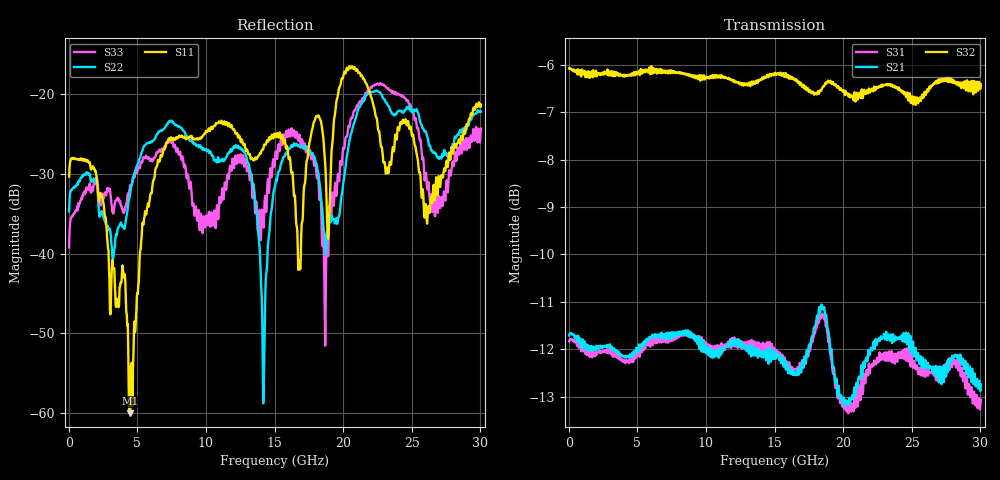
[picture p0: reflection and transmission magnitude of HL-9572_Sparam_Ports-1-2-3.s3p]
# GHZ S RI R 50.0
!; PortSelection: Port_123
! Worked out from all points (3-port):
!   858 points, 35 MHz to 30.03 GHz, reference 50 ohm
!   strongest paths, dB at 35 MHz, 7.525 GHz, 15.05 GHz, 22.54 GHz, 30.03 GHz:
!     S32: -6.1, -6.1, -6.2, -6.5, -6.4
!     S21: -11.7, -11.7, -12.2, -11.8, -12.7
!     S31: -11.8, -11.8, -12.1, -12.2, -13.1
!   lowest |S11| = -60.1 dB at 4.48 GHz (marker M1), VSWR 1.00, Z = 50.1 - j0.0158 ohm
!   |S11| at or under -10 dB: start of sweep to end of sweep
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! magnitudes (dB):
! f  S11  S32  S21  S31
! 35 MHz  -30.3  -6.1  -11.7  -11.8
! 4.48 GHz  -60.1  -6.2  -12.1  -12.2
! 7.175 GHz  -26.1  -6.1  -11.8  -11.7
! 12.85 GHz  -26.5  -6.4  -11.9  -11.9
! 14.18 GHz  -26.9  -6.3  -12.1  -12.0
! 15.05 GHz  -25.2  -6.2  -12.2  -12.1
! 16.8 GHz  -40.8  -6.4  -12.5  -12.4
! 18.76 GHz  -31.6  -6.4  -11.3  -11.5
! 20.37 GHz  -16.9  -6.6  -13.2  -13.4
! 30.03 GHz  -21.3  -6.4  -12.7  -13.1
